DATA_BLOCK "Parameter"
TITLE =
VERSION : 0.1


  STRUCT
   Activate : STRUCT
    Telegram0 : BOOL ;
    telegram1 : BOOL ;
    telegram2 : BOOL ;
    telegram3 : BOOL ;
   END_STRUCT ;
   telegram3 : STRUCT
    DisableMask : WORD ;
    InversionMask : WORD ;
   END_STRUCT ;
   telegram4 : STRUCT
    DisableMask : WORD ;
    InversionMask : WORD ;
   END_STRUCT ;
   telegram31 : STRUCT
    DisableMask : WORD ;
    InversionMask : WORD ;
   END_STRUCT ;
   telegram32 : STRUCT
    DisableMask : WORD ;
    InversionMask : WORD ;
   END_STRUCT ;
   telegram33 : STRUCT
    DisableMask : WORD ;
    InversionMask : WORD ;
   END_STRUCT ;
  END_STRUCT ;
BEGIN
   Activate.Telegram0 := FALSE;
   Activate.telegram1 := FALSE;
   Activate.telegram2 := FALSE;
   Activate.telegram3 := FALSE;
   telegram3.DisableMask := W#16#0;
   telegram3.InversionMask := W#16#0;
   telegram4.DisableMask := W#16#0;
   telegram4.InversionMask := W#16#0;
   telegram31.DisableMask := W#16#0;
   telegram31.InversionMask := W#16#0;
   telegram32.DisableMask := W#16#0;
   telegram32.InversionMask := W#16#0;
   telegram33.DisableMask := W#16#0;
   telegram33.InversionMask := W#16#0;
END_DATA_BLOCK

